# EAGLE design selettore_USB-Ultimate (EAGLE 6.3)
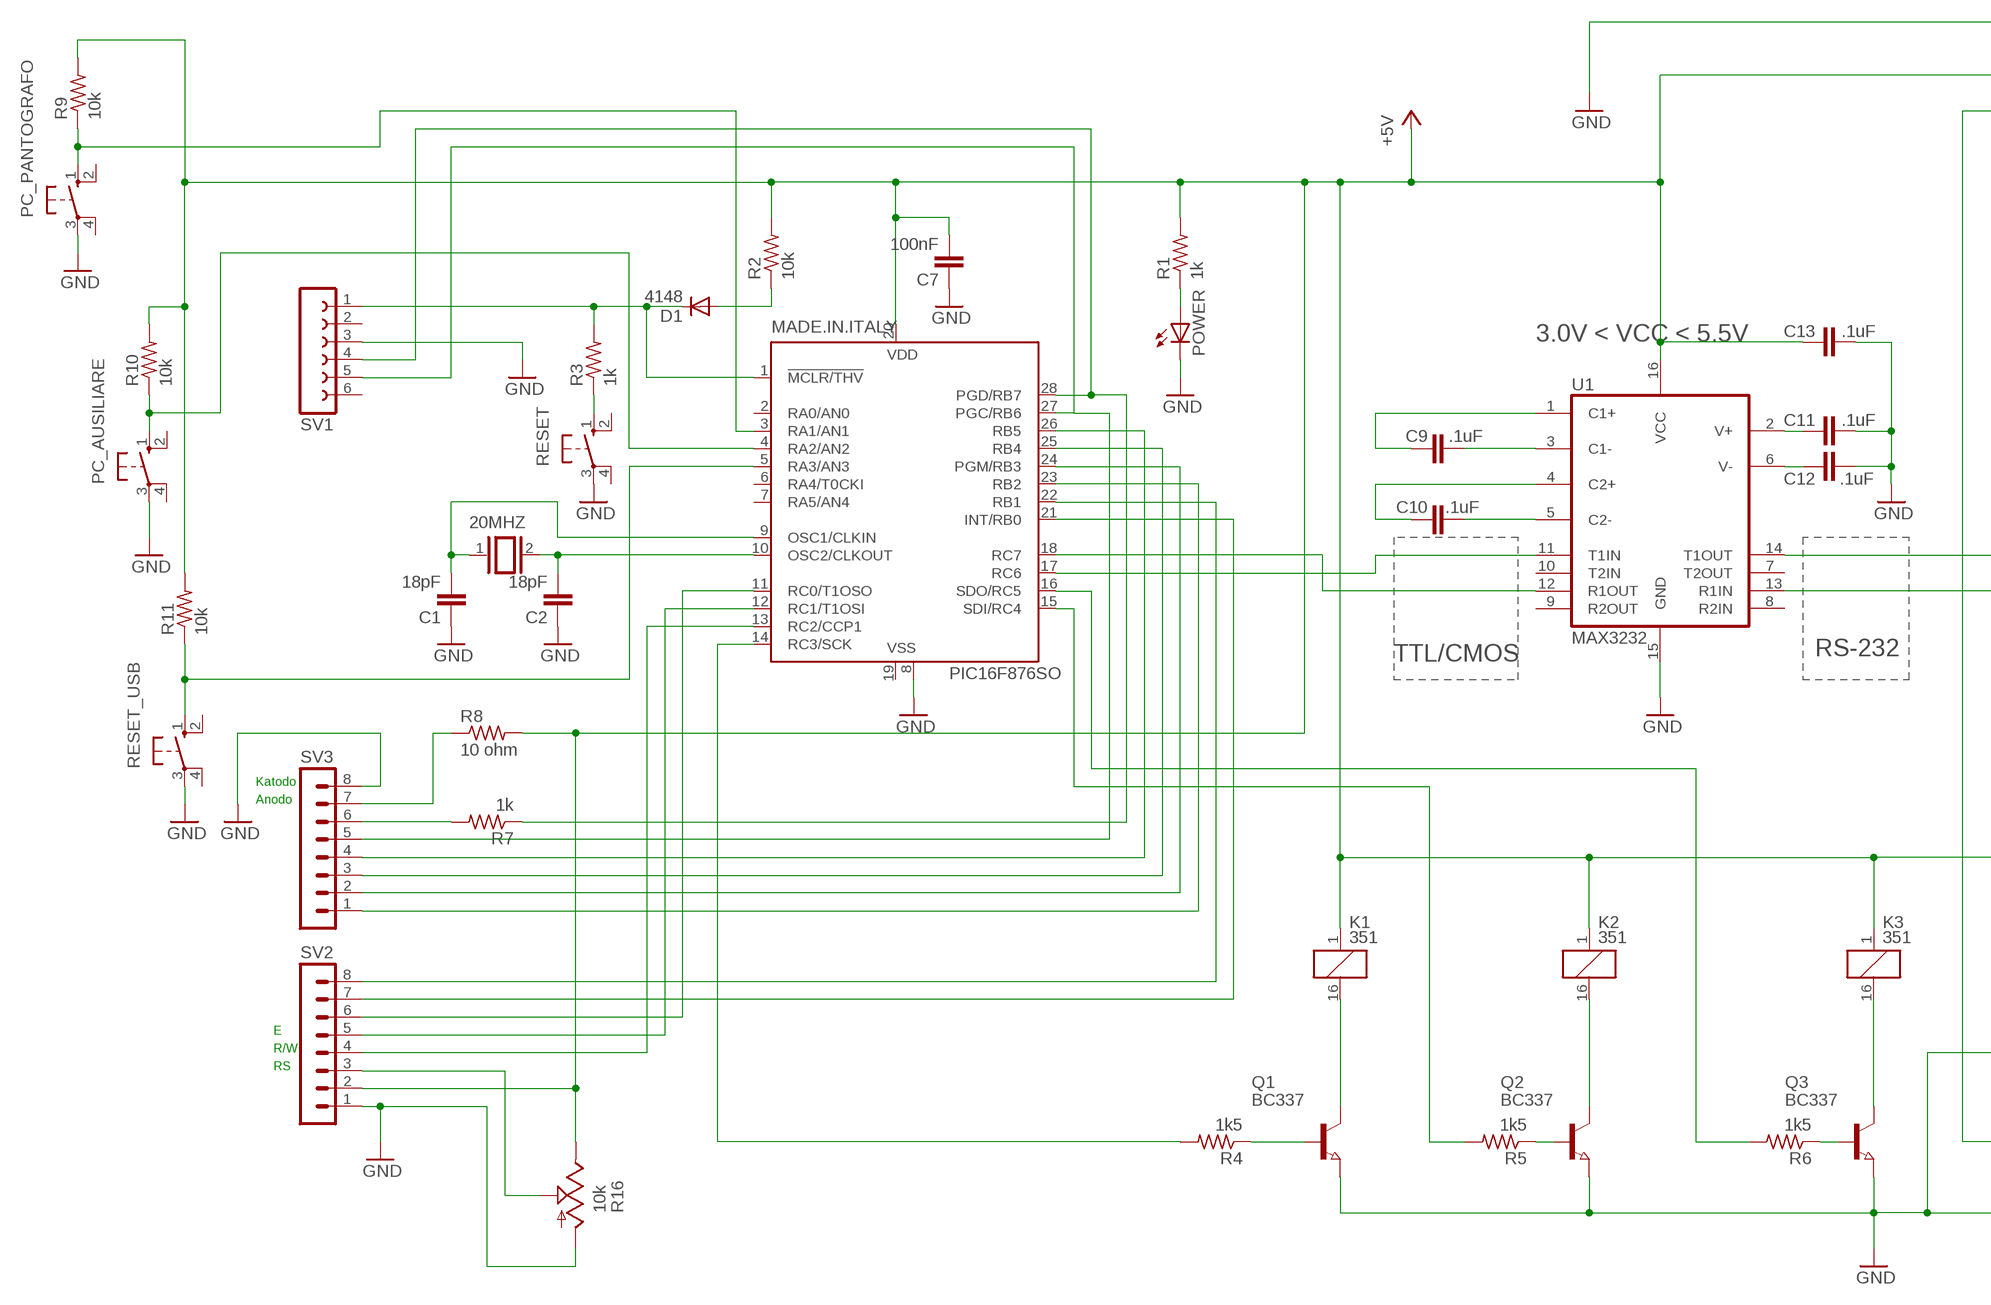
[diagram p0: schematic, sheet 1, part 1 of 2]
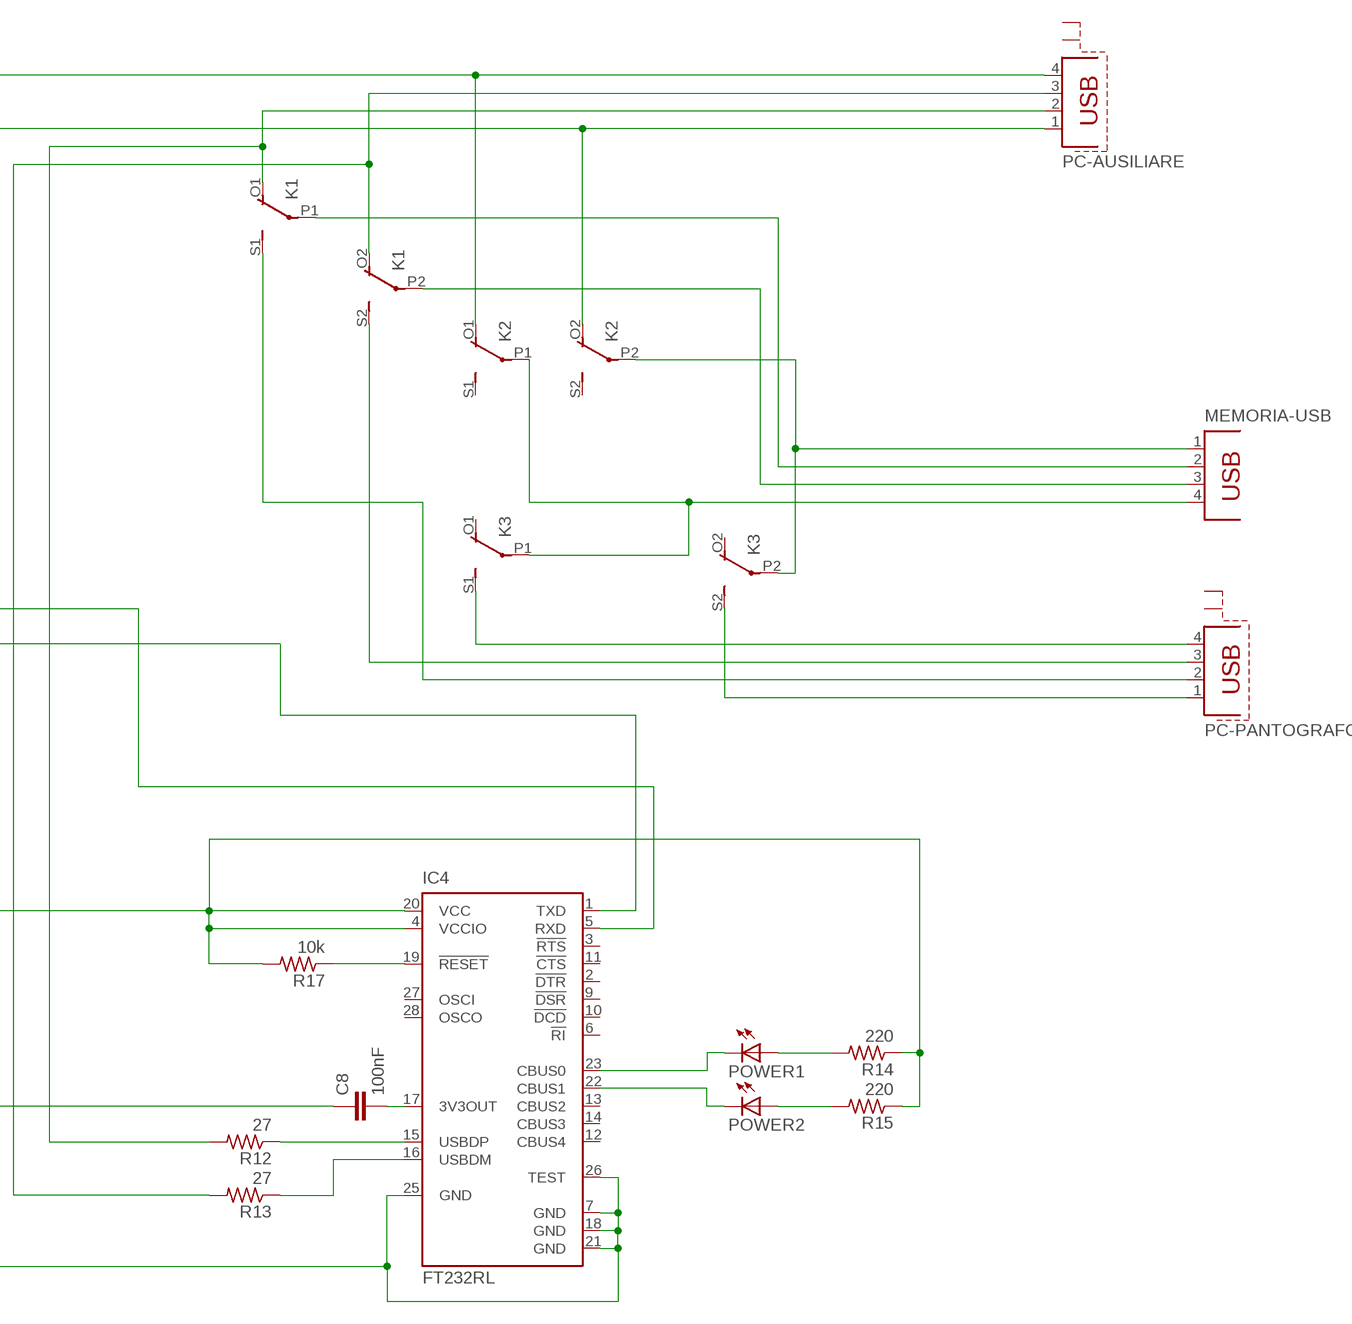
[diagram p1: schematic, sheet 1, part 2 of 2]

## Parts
20MHZ  XTAL/S  [QS]
C1  18pF  C-EUC0603  [C0603]
C2  18pF  C-EUC0603  [C0603]
C7  100nF  C-EUC0603  [C0603]
C8  100nF  C-EUC0603  [C0603]
C9  .1uF  CAP0402-CAP  [0402-CAP]
C10  .1uF  CAP0402-CAP  [0402-CAP]
C11  .1uF  CAP0402-CAP  [0402-CAP]
C12  .1uF  CAP0402-CAP  [0402-CAP]
C13  .1uF  CAP0402-CAP  [0402-CAP]
D1  4148  DIODE-DO214AC  [DO214AC]
IC4  FT232RL  [SSOP28]
K1  351  [351]
K2  351  [351]
K3  351  [351]
MADE.IN.ITALY  PIC16F876SO  [SO28W]
MEMORIA-USB  PN87520  [PN87520]
PC-AUSILIARE  PN61729-S  [PN61729-S]
PC-PANTOGRAFO  PN61729-S  [PN61729-S]
PC_AUSILIARE  10-XX  [B3F-10XX]
PC_PANTOGRAFO  10-XX  [B3F-10XX]
POWER  LED3MM  [LED3MM]
POWER1  LED3MM  [LED3MM]
POWER2  LED3MM  [LED3MM]
Q1  BC337  NPN-TRANSISTOR_SOT23  [SOT23]
Q2  BC337  NPN-TRANSISTOR_SOT23  [SOT23]
Q3  BC337  NPN-TRANSISTOR_SOT23  [SOT23]
R1  1k  R-US_M1206  [M1206]
R2  10k  R-US_M1206  [M1206]
R3  1k  R-US_M1206  [M1206]
R4  1k5  R-US_M1206  [M1206]
R5  1k5  R-US_M1206  [M1206]
R6  1k5  R-US_M1206  [M1206]
R7  1k  R-US_M1206  [M1206]
R8  10 ohm  R-US_M1206  [M1206]
R9  10k  R-US_M1206  [M1206]
R10  10k  R-US_M1206  [M1206]
R11  10k  R-US_M1206  [M1206]
R12  27  R-US_M1206  [M1206]
R13  27  R-US_M1206  [M1206]
R14  220  R-US_M1206  [M1206]
R15  220  R-US_M1206  [M1206]
R16  10k  TRIM_US-PT-10S  [PT-10S]
R17  10k  R-US_M1206  [M1206]
RESET  10-XX  [B3F-10XX]
RESET_USB  10-XX  [B3F-10XX]
SV1  FE06-1  [FE06]
SV2  MA08-1  [MA08-1]
SV3  MA08-1  [MA08-1]
U1  MAX3232  MAX232SOIC16  [SO016]

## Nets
4148: D1.A R2.1
+5V: C7.2 C13.1 IC4.4(VCCIO) IC4.20(VCC) K1.1 K2.1 K2.O2(3:O) K3.1 MADE.IN.ITALY.20(VDD) PC-AUSILIARE.1 R1.2 R2.2 R8.2 R9.2 R10.2 R11.2 R14.1 R15.1 R16.E R17.2 SV2.2 U1.16(VCC)
C1+: C9.1 U1.1(C1+)
C1-: C9.2 U1.3(C1-)
C2+: C10.1 U1.4(C2+)
C2-: C10.2 U1.5(C2-)
GND: C1.1 C2.1 C7.1 C8.1 C11.2 C12.2 C13.2 IC4.7(GND) IC4.18(GND) IC4.21(GND) IC4.25(GND) IC4.26(TEST) K2.O1(2:O) MADE.IN.ITALY.8(VSS) PC-AUSILIARE.4 PC_AUSILIARE.3(P) PC_PANTOGRAFO.3(P) POWER.K(C) Q1.2(E) Q2.2(E) Q3.2(E) R16.A RESET.3(P) RESET_USB.3(P) SV1.3 SV2.1 SV3.8 U1.15(GND)
N$1: IC4.15(USBDP) R12.1
N$2: MADE.IN.ITALY.4(RA2/AN2) PC_AUSILIARE.1(S) R10.1
N$3: IC4.16(USBDM) R13.1
N$4: IC4.19(!RESET) R17.1
N$5: IC4.23(CBUS0) POWER1.K(C)
N$6: IC4.22(CBUS1) POWER2.K(C)
N$7: K1.16 Q1.3(C)
N$8: K2.16 Q2.3(C)
N$9: K3.16 Q3.3(C)
N$10: MADE.IN.ITALY.14(RC3/SCK) R4.2
N$11: IC4.5(RXD) U1.14(T1OUT)
N$12: Q2.1(B) R5.1
N$13: Q3.1(B) R6.1
N$14: Q1.1(B) R4.1
N$15: MADE.IN.ITALY.15(SDI/RC4) R5.2
N$16: MADE.IN.ITALY.16(SDO/RC5) R6.2
N$18: MADE.IN.ITALY.18(RC7) U1.12(R1OUT)
N$20: POWER.A R1.1
N$21: K2.P2(3:P) K3.P2(3:P) MEMORIA-USB.1
N$22: R3.1 RESET.1(S)
N$23: D1.C MADE.IN.ITALY.1(!MCLR/THV) R3.2 SV1.1
N$24: K1.P1(2:P) MEMORIA-USB.2
N$26: 20MHZ.1 C1.2 MADE.IN.ITALY.9(OSC1/CLKIN)
N$27: 20MHZ.2 C2.2 MADE.IN.ITALY.10(OSC2/CLKOUT)
N$36: K1.P2(3:P) MEMORIA-USB.3
N$37: K1.O1(2:O) PC-AUSILIARE.2 R12.2
N$38: K1.S1(2:S) PC-PANTOGRAFO.2
N$39: K1.O2(3:O) PC-AUSILIARE.3 R13.2
N$40: K1.S2(3:S) PC-PANTOGRAFO.3
N$44: IC4.1(TXD) U1.13(R1IN)
N$45: MADE.IN.ITALY.27(PGC/RB6) SV1.5 SV3.5
N$46: MADE.IN.ITALY.28(PGD/RB7) R7.1 SV1.4
N$47: K2.P1(2:P) K3.P1(2:P) MEMORIA-USB.4
N$48: K3.S1(2:S) PC-PANTOGRAFO.4
N$49: POWER2.A R15.2
N$50: POWER1.A R14.2
N$52: C8.2 IC4.17(3V3OUT)
N$53: K3.S2(3:S) PC-PANTOGRAFO.1
N$54: R8.1 SV3.7
N$55: R7.2 SV3.6
N$56: MADE.IN.ITALY.26(RB5) SV3.4
N$57: MADE.IN.ITALY.25(RB4) SV3.3
N$58: MADE.IN.ITALY.24(PGM/RB3) SV3.2
N$59: MADE.IN.ITALY.23(RB2) SV3.1
N$60: MADE.IN.ITALY.22(RB1) SV2.8
N$62: MADE.IN.ITALY.11(RC0/T1OSO) SV2.6
N$63: MADE.IN.ITALY.12(RC1/T1OSI) SV2.5
N$64: MADE.IN.ITALY.13(RC2/CCP1) SV2.4
N$65: MADE.IN.ITALY.21(INT/RB0) SV2.7
N$66: MADE.IN.ITALY.5(RA3/AN3) R11.1 RESET_USB.1(S)
N$67: R16.S SV2.3
N$68: MADE.IN.ITALY.3(RA1/AN1) PC_PANTOGRAFO.1(S) R9.1
T1IN: MADE.IN.ITALY.17(RC6) U1.11(T1IN)
V+: C11.1 U1.2(V+)
V-: C12.1 U1.6(V-)
Unconnected: IC4.2(!DTR) IC4.3(!RTS) IC4.6(!RI) IC4.9(!DSR) IC4.10(!DCD) IC4.11(!CTS) IC4.12(CBUS4) IC4.13(CBUS2) IC4.14(CBUS3) IC4.27(OSCI) IC4.28(OSCO) K2.S1(2:S) K2.S2(3:S) K3.O1(2:O) K3.O2(3:O) MADE.IN.ITALY.2(RA0/AN0) MADE.IN.ITALY.6(RA4/T0CKI) MADE.IN.ITALY.7(RA5/AN4) PC-AUSILIARE.S1 PC-AUSILIARE.S2 PC-PANTOGRAFO.S1 PC-PANTOGRAFO.S2 PC_AUSILIARE.2(S1) PC_AUSILIARE.4(P1) PC_PANTOGRAFO.2(S1) PC_PANTOGRAFO.4(P1) RESET.2(S1) RESET.4(P1) RESET_USB.2(S1) RESET_USB.4(P1) SV1.2 SV1.6 U1.7(T2OUT) U1.8(R2IN) U1.9(R2OUT) U1.10(T2IN)

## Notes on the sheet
- 3.0V < VCC < 5.5V
- TTL/CMOS | RS-232
- Katodo
- Anodo
- E
- R/W
- RS

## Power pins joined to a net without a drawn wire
VSS: MADE.IN.ITALY.19(VSS)

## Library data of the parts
20MHZ = special:XTAL/S: CRYSTAL
C1 C2 C7 C8 = resistor:C-EU: CAPACITOR, European symbol
C9-C13 = SparkFun-Passives:CAP: Capacitor; PROD_ID: CAP-00810; SPARKLE_ID: 918
D1 = diode:DIODE-: DIODE
IC4 = ftdichip:FT232R: Source: http://www.ftdichip.com/Documents/DataSheets/DS_FT232R_v104.pdf; MPN: FT232RL; OC_FARNELL: 1146032; OC_NEWARK: 91K9918
K1-K3 = relay:351: RELAY 2 x switch, Omron; OC_FARNELL: unknown; OC_NEWARK: unknown
MADE.IN.ITALY = microchip:PIC16*876: MICROCONTROLLER flash type; MF: MICROCHIP; MPN: PIC16F876-20/SO; OC_FARNELL: 9761268; OC_NEWARK: 12C1950
MEMORIA-USB = con-berg:PN87520: BERG USB connector; OC_FARNELL: unknown; OC_NEWARK: unknown
PC-AUSILIARE PC-PANTOGRAFO = con-berg:PN61729-S: BERG USB connector; OC_FARNELL: unknown; OC_NEWARK: unknown
PC_AUSILIARE PC_PANTOGRAFO RESET RESET_USB = switch-omron:10-XX: OMRON SWITCH
POWER POWER1 POWER2 = led:LED: LED
Q1-Q3 = semicon-smd-ipc:NPN-TRANSISTOR_: NPN TRANSISTOR
R1-R15 R17 = resistor:R-US_: RESISTOR, American symbol
R16 = pot:TRIM_US-: POTENTIOMETER
SV1 = con-lsta:FE06-1: FEMALE HEADER
SV2 SV3 = con-lstb:MA08-1: PIN HEADER; OC_FARNELL: unknown; OC_NEWARK: unknown
U1 = SparkFun-DigitalIC:MAX232: RS232 Transceiver Very common IC. This is generically called 'MAX232', but works with the 3V equivalent MAX3232 generic ICs. Field tested and mother approved. Spark Fun Electronics SKU : COM-00316 (DIP) and COM-00589 (SMD); PROD_ID: IC-08171

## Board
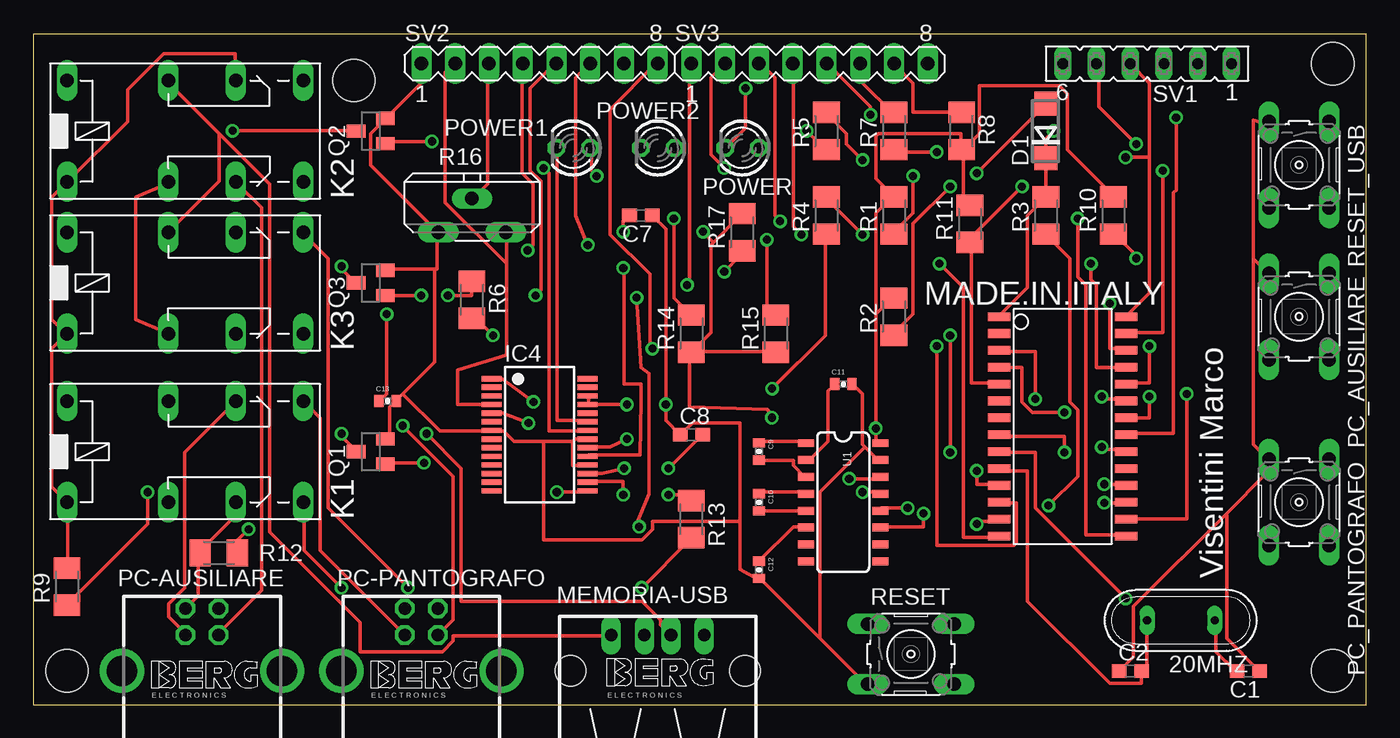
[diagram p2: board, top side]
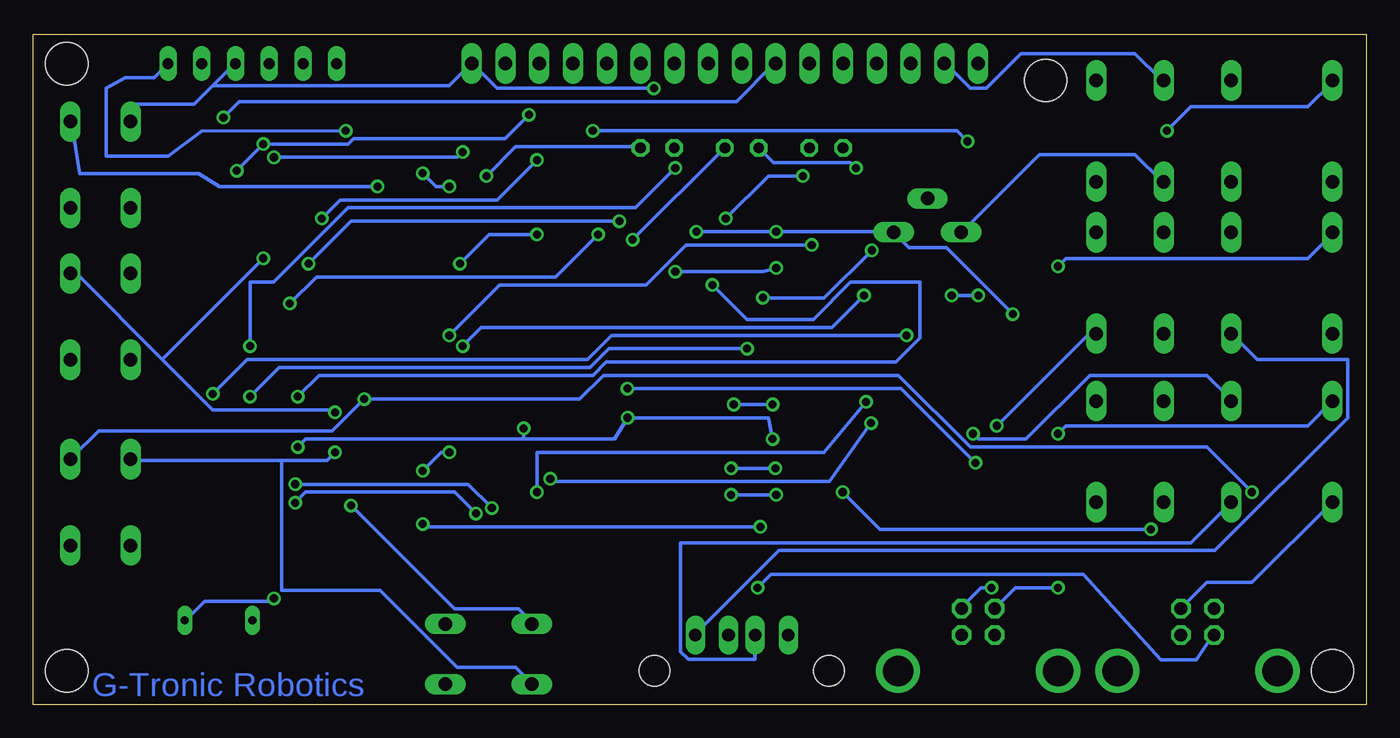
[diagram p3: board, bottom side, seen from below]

Size 100.31 x 50.47 mm. Coordinates in mm from the lower left corner, seen from the top.
Outline: 0,0 100.31,0 100.31,50.47 0,50.47 0,0
Copper layers (1*16): Top 0.035mm / dielectric 1.5mm / Bottom 0.035mm
Design rules "default": minimum track width 10mil, minimum drill 24mil, track to track 8mil, track to pad 8mil, pad to pad 8mil, via to via 8mil, smd to smd 8mil, copper to edge 40mil, drill to drill 8mil, minimum pad ring 10mil, minimum via ring 8mil, stop-mask expansion 4mil, vias tented up to drill 0mil, thermal gap 10mil
Holes 3.2 mm at 97.79,2.54 2.54,2.54 97.79,48.26 24.13,46.99

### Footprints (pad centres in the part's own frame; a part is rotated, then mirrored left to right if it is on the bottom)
QS = drill 0.61 long: 1 -2.54,0; 2 2.54,0
C0603 = smd 1.1 x 1: 1 -0.85,0; 2 0.85,0
0402-CAP = smd 0.7 x 0.9: 1 -0.65,0; 2 0.65,0
DO214AC = smd 1.8 x 1.7: A 2.05,0; C -2.05,0
SSOP28 = smd 0.4 x 1.5: 1 -4.225,-3.625; 2 -3.575,-3.625; 3 -2.925,-3.625; 4 -2.275,-3.625; 5 -1.625,-3.625; 6 -0.975,-3.625; 7 -0.325,-3.625; 8 0.325,-3.625; 9 0.975,-3.625; 10 1.625,-3.625; 11 2.275,-3.625; 12 2.925,-3.625; 13 3.575,-3.625; 14 4.225,-3.625; 15 4.225,3.625; 16 3.575,3.625; 17 2.925,3.625; 18 2.275,3.625; 19 1.625,3.625; 20 0.975,3.625; 21 0.325,3.625; 22 -0.325,3.625; 23 -0.975,3.625; 24 -1.625,3.625; 25 -2.275,3.625; 26 -2.925,3.625; 27 -3.575,3.625; 28 -4.225,3.625
351 = drill 1.016 long: 1 -3.81,-3.81; 16 -3.81,3.81; O1 8.89,-3.81; O2 8.89,3.81; P1 3.81,-3.81; P2 3.81,3.81; S1 13.97,-3.81; S2 13.97,3.81
SO28W = smd 0.65 x 1.7: 1 -7.62,-4.78; 2 -6.35,-4.78; 3 -5.08,-4.78; 4 -3.81,-4.78; 5 -2.54,-4.78; 6 -1.27,-4.78; 7 0,-4.78; 8 1.27,-4.78; 9 2.54,-4.78; 10 3.81,-4.78; 11 5.08,-4.78; 12 6.35,-4.78; 13 7.62,-4.78; 14 8.89,-4.78; 15 8.89,4.78; 16 7.62,4.78; 17 6.35,4.78; 18 5.08,4.78; 19 3.81,4.78; 20 2.54,4.78; 21 1.27,4.78; 22 0,4.78; 23 -1.27,4.78; 24 -2.54,4.78; 25 -3.81,4.78; 26 -5.08,4.78; 27 -6.35,4.78; 28 -7.62,4.78
PN87520 = drill 0.95 long: 1 -3.5,2.71; 2 -1,2.71; 3 1,2.71; 4 3.5,2.71 | hole 2.3: -6.57,0; 6.57,0
PN61729-S = drill 0.95 octagon: 1 1.25,4.71; 2 -1.25,4.71; 3 -1.25,2.71; 4 1.25,2.71 | drill 2.3 pad 2.9: S1 -6.02,0; S2 6.02,0
B3F-10XX = drill 1.016 long: 1 -3.251,2.261; 2 3.251,2.261; 3 -3.251,-2.261; 4 3.251,-2.261
LED3MM = drill 0.813 octagon: A -1.27,0; K 1.27,0
SOT23 = smd 1 x 1.4: 1 -0.95,-1.1; 2 0.95,-1.1; 3 0,1.1
M1206 = smd 1.6 x 2: 1 -1.4,0; 2 1.4,0
PT-10S = drill 1.016 long: A -2.54,-1.27; E 2.54,-1.27; S 0,1.27
FE06 = drill 0.813 long: 1 -6.35,0; 2 -3.81,0; 3 -1.27,0; 4 1.27,0; 5 3.81,0; 6 6.35,0
MA08-1 = drill 1.016 long: 1 -8.89,0; 2 -6.35,0; 3 -3.81,0; 4 -1.27,0; 5 1.27,0; 6 3.81,0; 7 6.35,0; 8 8.89,0
SO016 = smd 0.6 x 1.2: 1 -4.445,-2.8; 2 -3.175,-2.8; 3 -1.905,-2.8; 4 -0.635,-2.8; 5 0.635,-2.8; 6 1.905,-2.8; 7 3.175,-2.8; 8 4.445,-2.8; 9 4.445,2.8; 10 3.175,2.8; 11 1.905,2.8; 12 0.635,2.8; 13 -0.635,2.8; 14 -1.905,2.8; 15 -3.175,2.8; 16 -4.445,2.8

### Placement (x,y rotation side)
20MHZ  86.36,6.35 180 top
C1  91.44,2.54 180 top
C2  82.55,2.54 0 top
C7  45.72,36.83 180 top
C8  49.53,20.32 0 top
C9  54.61,19.05 270 top
C10  54.61,15.24 270 top
C11  60.96,24.13 0 top
C12  54.61,10.16 270 top
C13  26.67,22.86 0 top
D1  76.2,43.18 90 top
IC4  38.1,20.32 270 top
K1  6.35,19.05 0 top
K2  6.35,43.18 0 top
K3  6.35,31.75 0 top
MADE.IN.ITALY  77.47,21.59 270 top
MEMORIA-USB  46.99,2.54 0 top
PC-AUSILIARE  12.7,2.54 0 top
PC-PANTOGRAFO  29.21,2.54 0 top
PC_AUSILIARE  95.25,29.21 270 top
PC_PANTOGRAFO  95.25,15.24 270 top
POWER  53.34,41.91 180 top
POWER1  40.64,41.91 180 top
POWER2  46.99,41.91 180 top
Q1  25.4,19.05 90 top
Q2  25.4,43.18 90 top
Q3  25.4,31.75 90 top
R1  64.77,36.83 90 top
R2  64.77,29.21 90 top
R3  76.2,36.83 90 top
R4  59.69,36.83 90 top
R5  59.69,43.18 90 top
R6  33.02,30.48 270 top
R7  64.77,43.18 90 top
R8  69.85,43.18 270 top
R9  2.54,8.89 90 top
R10  81.28,36.83 90 top
R11  70.48,36.2 90 top
R12  13.97,11.43 180 top
R13  49.53,13.97 270 top
R14  49.53,27.94 90 top
R15  55.88,27.94 90 top
R16  33.02,36.83 0 top
R17  53.34,35.56 90 top
RESET  66.04,3.81 0 top
RESET_USB  95.25,40.64 270 top
SV1  83.82,48.26 180 top
SV2  38.1,48.26 0 top
SV3  58.42,48.26 0 top
U1  60.96,15.24 270 top

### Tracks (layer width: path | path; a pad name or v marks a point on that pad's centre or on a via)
4148  (via drill 0.61)
  Top 0.254: v71,40 76.2,45.2 D1.A | v69,39 66.2,36.2 66.2,29.4 64.8,28 R2.1
  Bottom 0.254: v71,40 70,39 v69,39
+5V  (via drill 0.61)
  Top 0.254: 63.4,29.4 v63.4,20.8 63.4,20 63.6,19.8 U1.16 | 63.4,29.4 64.6,30.6 R2.2 | 63.4,29.4 63.4,37 64.6,38.2 R1.2 63.4,39.6 63.4,42.8 63.6,43 69.8,43 69.8,41.8 R8.2 | R11.2 70.4,37.6 70,38 70,41.6 R8.2 | R10.2 81.2,38.4 77.8,41.8 77.8,46 77.2,46.6 71.2,46.6 71.2,43 70,41.8 R8.2 | v44.67,20 43.4,19.4 41.8,19.4 IC4.20 | v55.59,21.6 55.24,22.23 49.4,22.4 49.4,26.4 R14.1 49.6,26.6 | v80.4,19.4 80.4,19.2 82.2,19.2 MADE.IN.ITALY.20 | 51.2,34.8 51,34.6 51,28 49.6,26.6 | 51.2,34.8 53.2,36.8 R17.2 | 49.6,26.6 55.8,26.6 R15.1 | R9.2 2.6,10.4 2.6,15.2 K1.1 2.4,15.4 1.4,16.4 1.4,26.8 K3.1 2.4,28 1.4,29 1.4,38.2 2.4,39.2 K2.1 2.6,39.4 7.09,43.9 7.09,46.3 9.8,49 15.2,49 15.2,47 K2.O2 | v26.6,29.4 26.6,23.4 26.2,23 C13.1 | v44.4,35.6 44.4,36.4 44.8,36.8 C7.2 | 35.6,33.2 35.6,35.4 R16.E | 35.6,33.2 35.6,26.33 31.93,25.2 31.93,22.6 34.4,22.6 IC4.4 | 35.6,33.2 31,37.8 31,47.6 31.6,48.2 SV2.2 | v50.4,35.6 51.2,34.8
  Bottom 0.254: v44.67,20 45,21.6 v55.59,21.6 56.55,20 63.4,20 | v80.4,19.4 79.8,20 63.4,20 | 63.4,20 v63.4,20.8 | PC-AUSILIARE.1 12,9.2 8.6,9.2 2.6,15.2 K1.1 | K2.O2 15.4,47 17.4,49 26,49 28.6,46.4 29.8,46.4 31.6,48.2 SV2.2 | v26.6,29.4 31.6,34.4 34.4,34.4 R16.E 35.6,35.6 v44.4,35.6 v50.4,35.6
C1+
  Top 0.254: C9.1 54.8,19.8 58,19.8 U1.1
C1-
  Top 0.254: C9.2 57.2,18.4 57.2,18 58,17.2 U1.3
C2+
  Top 0.254: C10.1 54.8,16 58,16 U1.4
C2-
  Top 0.254: C10.2 54.8,14.6 58,14.6 U1.5
GND  (via drill 0.61)
  Top 0.254: 89.8,14.4 92.8,17.4 92.8,18.4 PC_PANTOGRAFO.3 92.8,18.6 91.8,19.6 91.8,33.6 | 89.8,14.4 82.8,7.4 82.8,3.6 81.8,2.6 C2.1 | 89.8,14.4 89.8,5 92.2,2.6 C1.1 | v77.6,19 77.6,20.2 72.8,20.2 MADE.IN.ITALY.8 | v53.6,46.4 53.6,43.4 52.2,42 POWER.K | 91.8,33.6 92.8,32.6 PC_AUSILIARE.3 | 91.8,33.6 91.8,44 92.8,43.73 RESET_USB.3 | 41.8,22.6 41.8,23.2 IC4.26 | C7.1 47.6,35.8 v47.6,22.6 47.6,21.4 C8.1 48.8,20.4 49.6,21.2 53.16,21.2 53.16,13.8 | v44.67,22.6 41.8,22.6 | 41.8,22.6 IC4.25 | 62.6,19.4 63.6,18.4 U1.15 | 62.6,19.4 62.4,19.6 62.4,23.4 61.8,24 C11.2 | 59.2,5 62.6,1.6 RESET.3 | 59.2,5 54.8,9.4 C12.2 54.6,9.4 53.16,10.2 53.16,13.8 | 62.6,19.4 59.2,16 59.2,5 | PC-AUSILIARE.4 14,5.4 17.2,8.6 17.2,37.4 15.4,39.2 K2.O1 | 40.6,19.8 40.6,18 41.6,18 IC4.18 | 40.6,19.8 40.8,20 41.6,20 IC4.21 | 40.6,19.8 38.4,19.8 | 38.4,19.8 36.2,19.8 35.4,20.6 34.6,20.6 IC4.7 34.4,20.6 30.6,20.6 27.8,23.4 | SV2.1 29.2,48.2 29.2,46.8 26.6,44.2 Q2.2 26.4,44 25.4,43 25.4,40.6 30.4,35.6 R16.A 30.4,35.4 30.4,32.8 30.2,32.8 | Q1.2 26.6,20 26.8,20.2 26.8,22.4 27.2,22.8 C13.2 27.4,23 27.8,23.4 | 30.2,32.8 26.6,32.8 Q3.2 | 27.8,23.4 30.2,25.8 30.2,32.8 | 53.16,13.8 46.6,13.8 46.6,13.2 45.8,12.4 38.4,12.4 38.4,19.8
  Bottom 0.254: v77.6,19 78.2,18.4 81.6,18.4 | 81.6,18.4 92.8,18.4 PC_PANTOGRAFO.3 | v53.6,46.4 65.4,46.4 67.2,48.2 SV3.8 67.4,48.2 69,46.6 86.8,46.6 | 86.8,46.6 88.2,45.2 92.8,45.2 RESET_USB.3 | 86.8,46.6 85.2,48.2 SV1.3 | v47.6,22.6 v44.67,22.6 | K2.O1 15.4,39.4 17.4,41.4 24.6,41.4 30.4,35.6 R16.A | 81.6,18.4 81.6,8.6 74.2,8.6 68.4,2.8 64,2.8 62.8,1.6 RESET.3
N$1  (via drill 0.61)
  Top 0.254: v39.4,16 41.6,16 IC4.15 | v16.2,13.2 15.4,12.4 15.4,11.6 R12.1
  Bottom 0.254: v39.4,16 36.6,13.2 v16.2,13.2
N$2  (via drill 0.61)
  Top 0.254: MADE.IN.ITALY.4 74.4,25.4 74.4,22.8 75.2,22 v77.6,22 | v83,33.6 83,33.8 81.4,35.4 R10.1
  Bottom 0.254: v77.6,22 77.8,22.2 86.8,22.2 90.6,26 | 90.6,26 97,32.4 97.4,32.4 PC_AUSILIARE.1 | 90.6,26 v83,33.6
N$3  (via drill 0.61)
  Top 0.254: v44.4,15.8 44.4,16.8 41.8,16.8 IC4.16 | v47.8,15.8 49.4,15.8 49.4,15.4 R13.1
  Bottom 0.254: v47.8,15.8 v44.4,15.8
N$4  (via drill 0.61)
  Top 0.254: v44.4,32.87 44.45,32.87 44.45,24.13 45.72,24.13 45.72,22.86 45.67,18.8 41.8,18.8 IC4.19 | v52,32.6 53.2,33.8 53.2,34 R17.1
  Bottom 0.254: v44.4,32.87 45.4,32.6 v52,32.6
N$5
  Top 0.254: IC4.23 41.6,21.4 39.4,21.4 39.4,41.8 POWER1.K
N$6  (via drill 0.61)
  Top 0.254: v38.4,40.4 38.8,40 38.8,20.6 41.6,20.6 IC4.22
  Bottom 0.254: v38.4,40.4 38.8,40.8 44.6,40.8 45.6,41.8 POWER2.K
N$7  (via drill 0.61)
  Top 0.254: v23.2,20.4 23.2,20.2 24.2,19.2 Q1.3
  Bottom 0.254: v23.2,20.4 22.6,21 4.4,21 K1.16
N$8  (via drill 0.61)
  Top 0.254: v15,43.2 24.2,43.2 Q2.3
  Bottom 0.254: v15,43.2 13.2,45 4.4,45 2.6,46.8 K2.16
N$9  (via drill 0.61)
  Top 0.254: v23.2,33 23.2,32.8 24.2,31.8 Q3.3
  Bottom 0.254: v23.2,33 22.6,33.6 4.4,33.6 2.6,35.4 K3.16
N$10  (via drill 0.61)
  Top 0.254: v68.2,33.2 70,31.4 70,12.6 72.6,12.6 MADE.IN.ITALY.14 | v62.4,35.4 59.8,38 59.8,38.2 R4.2
  Bottom 0.254: v68.2,33.2 66,35.4 v62.4,35.4
N$11  (via drill 0.61)
  Top 0.254: v61.4,17 63.6,17 U1.14 | v37.27,21.2 35.2,22 34.6,22 IC4.5
  Bottom 0.254: v61.4,17 61.2,16.8 40.4,16.8 v37.27,21.2
N$12  (via drill 0.61)
  Top 0.254: v30,42.4 26.6,42.4 Q2.1 | v58.2,43.2 59.6,41.8 R5.1
  Bottom 0.254: v30,42.4 30.8,43.2 v58.2,43.2
N$13  (via drill 0.61)
  Top 0.254: v29.2,30.8 Q3.1 | v31.2,30.8 33,30.8 33,31.8 R6.1
  Bottom 0.254: v31.2,30.8 v29.2,30.8
N$14  (via drill 0.61)
  Top 0.254: v29.4,18.2 26.6,18.2 Q1.1 | v55.6,23.8 59.6,27.8 59.6,35.4 R4.1
  Bottom 0.254: v29.4,18.2 35,23.8 v55.6,23.8
N$15  (via drill 0.61)
  Top 0.254: v78.6,36.6 78.6,32.2 79.2,31.6 79.2,12.8 82.2,12.8 MADE.IN.ITALY.15 | v62.4,41 61.2,42.2 61.2,43 59.8,44.4 R5.2
  Bottom 0.254: v78.6,36.6 77.2,38 65.4,38 v62.4,41
N$16  (via drill 0.61)
  Top 0.254: v86.8,23.4 86.8,14 82.4,14 MADE.IN.ITALY.16 | v34.6,27.8 33.2,29.2 R6.2
  Bottom 0.254: v86.8,23.4 84.2,26 58.6,26 56.8,27.8 v34.6,27.8
N$18  (via drill 0.61)
  Top 0.254: v65.8,14.8 63.8,14.8 U1.12 | v80.6,16.6 82.2,16.6 MADE.IN.ITALY.18
  Bottom 0.254: v65.8,14.8 67.6,16.6 v80.6,16.6
N$20  (via drill 0.61)
  Top 0.254: v66.2,39.8 66.2,37 64.8,35.6 R1.1
  Bottom 0.254: v66.2,39.8 64,42 54.8,42 POWER.A
N$21
  Top 0.254: 14,43 10.2,46.8 K2.P2 | 14,43 17.8,39.2 17.8,13 24.6,6.2 24.6,4 30.8,4 31.6,4.8 31.6,5.2 43.4,5.2 MEMORIA-USB.1 | K3.P2 14,39.4 14,43
N$22  (via drill 0.61)
  Top 0.254: v76.4,15 78.6,17.2 78.6,22.2 78,22.8 78,33.6 76.2,35.4 R3.1
  Bottom 0.254: v76.4,15 68.6,7.2 63.8,7.2 62.8,6.2 RESET.1
N$23  (via drill 0.61)
  Top 0.254: MADE.IN.ITALY.1 72.8,29.4 74.8,31.4 74.8,36.8 76.2,38.2 R3.2 D1.C 76.2,42.6 v76.8,43.2
  Bottom 0.254: v76.8,43.2 87.63,43.18 90.17,41.3 94.83,41.3 94.83,46.4 93.4,47.2 91.2,47.2 90.2,48.2 SV1.1
N$24
  Bottom 0.254: K1.P1 13.2,12.2 51.6,12.2 51.6,4 51,3.4 46,3.4 46,5.2 MEMORIA-USB.2
N$26  (via drill 0.61)
  Top 0.254: C1.2 90.4,2.6 89,4 89,6.2 20MHZ.1 | v82.2,8 75.4,14.8 75.4,19 72.8,19 MADE.IN.ITALY.9
  Bottom 0.254: v82.2,8 82.4,7.8 87.4,7.8 88.8,6.4 20MHZ.1
N$27
  Top 0.254: 20MHZ.2 83.8,6.2 83.8,3 83.4,2.6 C2.2 83.4,1.6 81,1.6 74.8,7.8 74.8,17.6 72.8,17.6 MADE.IN.ITALY.10
N$36  (via drill 0.61)
  Top 0.254: v29.6,20.4 32.2,17.8 32.2,7.8 45.8,7.8 47.2,6.4 47.2,6 47.8,5.4 MEMORIA-USB.3
  Bottom 0.254: v29.6,20.4 29.2,20 25.6,20 20.8,24.8 12,24.8 10.2,23 K1.P2
N$37
  Top 0.254: K1.O1 15.2,15.2 15.2,14.2 12.6,11.6 R12.2 12.4,11.4 12.4,8.2 PC-AUSILIARE.2
N$38  (via drill 0.61)
  Top 0.254: v23.2,8.8 20.4,11.6 20.4,15.2 K1.S1
  Bottom 0.254: v23.2,8.8 26.4,8.8 27.8,7.4 PC-PANTOGRAFO.2
N$39  (via drill 0.61)
  Top 0.254: v45.8,8.8 49.4,12.4 R13.2 | K1.O2 15.2,22.8 11.4,19 11.4,8.8 10.2,7.6 10.2,6.6 11.4,5.4 PC-AUSILIARE.3
  Bottom 0.254: v45.8,8.8 44.8,9.8 21.27,9.8 15.47,3.37 12.8,3.37 11.6,5.2 PC-AUSILIARE.3
N$40
  Top 0.254: PC-PANTOGRAFO.3 27.8,5.4 21.6,11.6 21.6,21.6 20.4,22.8 K1.S2
N$44  (via drill 0.61)
  Top 0.254: v62.4,16 63.6,16 U1.13 | v37.63,22.8 35.2,24.6 34.6,24.6 IC4.1
  Bottom 0.254: v62.4,16 62.4,19 40.8,19 v37.63,22.8
N$45  (via drill 0.61)
  Top 0.254: v85,40.2 85,28 82.4,28 MADE.IN.ITALY.27 | v83,42.2 80.2,45 80.2,48.2 SV1.5 | v63,44.4 63,45 59.8,48.2 SV3.5
  Bottom 0.254: v85,40.2 v83,42.2 76.6,42.2 76.2,42.6 64.8,42.6 v63,44.4
N$46  (via drill 0.61)
  Top 0.254: 84,41.2 84,46.8 82.6,48.2 SV1.4 | 84,41.2 84,31 82.4,29.4 MADE.IN.ITALY.28 | v68,41.6 64.8,41.6 R7.1 | 84,41.2 v82.2,41.2
  Bottom 0.254: v68,41.6 68.4,41.2 v82.2,41.2
N$47
  Top 0.254: K2.P1 10,39.2 7.73,38.2 7.73,29 10,28 K3.P1
  Bottom 0.254: MEMORIA-USB.4 50.4,5.4 44.2,11.6 11.4,11.6 1.4,21.6 1.4,26 8.2,26 10,27.8 K3.P1
N$48  (via drill 0.61)
  Top 0.254: v27.8,21 31.6,17.2 31.6,6.4 30.6,5.4 PC-PANTOGRAFO.4
  Bottom 0.254: v27.8,21 21,27.8 20.4,27.8 K3.S1
N$49  (via drill 0.61)
  Top 0.254: v55.2,35 55.2,30 55.8,29.4 R15.2
  Bottom 0.254: v55.2,35 48.4,41.8 POWER2.A
N$50  (via drill 0.61)
  Top 0.254: v48.2,36.6 48.2,30.6 49.4,29.4 R14.2 | v42.4,39.8 42,40.2 42,41.8 POWER1.A
  Bottom 0.254: v48.2,36.6 45,39.8 v42.4,39.8
N$52  (via drill 0.61)
  Top 0.254: v47.8,17.8 50.2,20.2 C8.2 | v44.47,17.8 42.8,17.4 41.8,17.4 IC4.17
  Bottom 0.254: v44.47,17.8 v47.8,17.8
N$53  (via drill 0.61)
  Top 0.254: v28.2,8.8 22.2,14.8 22.2,33.6 20.4,35.4 K3.S2
  Bottom 0.254: v28.2,8.8 29,8.8 30.4,7.4 PC-PANTOGRAFO.1
N$54
  Top 0.254: R8.1 69.8,44.6 66.2,44.6 66.2,46.8 64.8,48.2 SV3.7
N$55
  Top 0.254: R7.2 64.6,44.6 62.4,46.8 62.4,48.2 SV3.6
N$56  (via drill 0.61)
  Top 0.254: v81,30.2 81,26.8 82.2,26.8 MADE.IN.ITALY.26 | v57.8,35.4 57.2,36 57.2,48.2 SV3.4
  Bottom 0.254: v81,30.2 79,32.2 61,32.2 v57.8,35.4
N$57  (via drill 0.61)
  Top 0.254: MADE.IN.ITALY.25 80,25.4 80,31.6 79.6,32 v79.6,33.2 | v56.2,36.4 55.8,36.8 55.8,47.2 54.8,48.2 SV3.3
  Bottom 0.254: v79.6,33.2 76.4,36.4 v56.2,36.4
N$58  (via drill 0.61)
  Top 0.254: v84,27 84,24.2 82.4,24.2 MADE.IN.ITALY.24 | v52,40.4 51,41.4 51,47.2 52,48.2 SV3.2
  Bottom 0.254: v84,27 84,31.8 82.2,31.8 76.6,37.4 55,37.4 v52,40.4
N$59  (via drill 0.61)
  Top 0.254: v80.4,23.2 80.4,23 82.2,23 MADE.IN.ITALY.23 | v49.2,31.6 49.4,31.8 49.4,48.2 SV3.1
  Bottom 0.254: v80.4,23.2 78.8,24.8 58.2,24.8 57.2,25.8 35.4,25.8 33.6,27.6 33.6,31.8 38.8,31.8 41.6,29 46.6,29 v49.2,31.6
N$60  (via drill 0.61)
  Top 0.254: v84,23.2 84,21.6 82.4,21.6 MADE.IN.ITALY.22 | v46.6,26.8 46.4,27 46.4,32.4 43.4,35.4 43.4,44.8 46.8,48.2 SV2.8
  Bottom 0.254: v84,23.2 81.8,25.4 58.4,25.4 57,26.8 v46.6,26.8
N$62  (via drill 0.61)
  Top 0.254: v71,17.6 71,16.6 72.6,16.6 MADE.IN.ITALY.11 | v69,27.8 v69,19 | v41.73,34.6 40.8,36.8 40.8,47.2 41.8,48.2 SV2.6
  Bottom 0.254: v71,17.6 69.6,19 v69,19 | v69,27.8 65.2,31.6 54.2,31.6 51.2,34.6 v41.73,34.6
N$63  (via drill 0.61)
  Top 0.254: v68,27 68,12 73.8,12 74,12.2 74,15.2 72.8,15.2 MADE.IN.ITALY.12 | v37.8,30.8 38.2,31.2 38.2,39.4 37.4,40.2 37.4,46.4 39.2,48.2 SV2.5
  Bottom 0.254: v68,27 66.6,28.4 40.2,28.4 v37.8,30.8
N$64  (via drill 0.61)
  Top 0.254: v71,13.6 71,13.8 72.6,13.8 MADE.IN.ITALY.13 | v45.6,13.4 45.4,13.6 46.35,15.88 46.35,24.92 45.72,25.4 v45.4,30.64 | v37.2,34.2 37.6,34.6 37.6,39.2 36.8,40 36.8,48.2 SV2.4
  Bottom 0.254: v71,13.6 70.8,13.4 v45.6,13.4 | v45.4,30.64 44.8,30.6 40.8,30.6 v37.2,34.2
N$65  (via drill 0.61)
  Top 0.254: v86,44.2 86,38.73 85.8,38.53 85.8,20.4 82.4,20.4 MADE.IN.ITALY.21
  Bottom 0.254: v86,44.2 84.8,45.4 47.4,45.4 44.6,48.2 SV2.7
N$66  (via drill 0.61)
  Top 0.254: MADE.IN.ITALY.5 72.6,24.2 70.6,24.2 70.6,34.6 R11.1 70.6,34.8 70.6,35.2 v74.4,39
  Bottom 0.254: v74.4,39 86.27,39 87.87,39.97 96.81,39.97 97.4,43.73 RESET_USB.1
N$67
  Top 0.254: R16.S 33.2,38.2 34.2,39.2 34.2,48.2 SV2.3
N$68  (via drill 0.61)
  Top 0.254: v75.4,23 75.4,26.6 72.8,26.6 MADE.IN.ITALY.3 | v8.6,16 8.6,13.6 2.6,7.6 R9.1
  Bottom 0.254: PC_PANTOGRAFO.1 97.4,18.6 95.4,20.6 77.8,20.6 v75.4,23 59.2,23 57.4,24.8 35.2,24.8 29.8,19.4 12,19.4 v8.6,16
T1IN  (via drill 0.61)
  Top 0.254: v67,14.4 67,13.4 63.8,13.4 U1.11 | v80.6,15.2 82.2,15.2 MADE.IN.ITALY.17
  Bottom 0.254: v67,14.4 68.6,16 79.8,16 v80.6,15.2
V+
  Top 0.254: C11.1 60.2,24 59.8,23.6 59.8,19.8 58.6,18.6 58.2,18.6 U1.2
V-
  Top 0.254: C12.1 57.2,13.4 58,13.4 U1.6

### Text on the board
Bottom: G-Tronic Robotics
tNames: Visentini Marco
